DATA_BLOCK DB 10
VERSION : 0.1


  STRUCT
   Daten : ARRAY  [0 .. 255 ] OF BYTE ;
  END_STRUCT ;
BEGIN
   Daten[0] := B#16#0;
   Daten[1] := B#16#0;
   Daten[2] := B#16#0;
   Daten[3] := B#16#0;
   Daten[4] := B#16#0;
   Daten[5] := B#16#0;
   Daten[6] := B#16#0;
   Daten[7] := B#16#0;
   Daten[8] := B#16#0;
   Daten[9] := B#16#0;
   Daten[10] := B#16#0;
   Daten[11] := B#16#0;
   Daten[12] := B#16#0;
   Daten[13] := B#16#0;
   Daten[14] := B#16#0;
   Daten[15] := B#16#0;
   Daten[16] := B#16#0;
   Daten[17] := B#16#0;
   Daten[18] := B#16#0;
   Daten[19] := B#16#0;
   Daten[20] := B#16#0;
   Daten[21] := B#16#0;
   Daten[22] := B#16#0;
   Daten[23] := B#16#0;
   Daten[24] := B#16#0;
   Daten[25] := B#16#0;
   Daten[26] := B#16#0;
   Daten[27] := B#16#0;
   Daten[28] := B#16#0;
   Daten[29] := B#16#0;
   Daten[30] := B#16#0;
   Daten[31] := B#16#0;
   Daten[32] := B#16#0;
   Daten[33] := B#16#0;
   Daten[34] := B#16#0;
   Daten[35] := B#16#0;
   Daten[36] := B#16#0;
   Daten[37] := B#16#0;
   Daten[38] := B#16#0;
   Daten[39] := B#16#0;
   Daten[40] := B#16#0;
   Daten[41] := B#16#0;
   Daten[42] := B#16#0;
   Daten[43] := B#16#0;
   Daten[44] := B#16#0;
   Daten[45] := B#16#0;
   Daten[46] := B#16#0;
   Daten[47] := B#16#0;
   Daten[48] := B#16#0;
   Daten[49] := B#16#0;
   Daten[50] := B#16#0;
   Daten[51] := B#16#0;
   Daten[52] := B#16#0;
   Daten[53] := B#16#0;
   Daten[54] := B#16#0;
   Daten[55] := B#16#0;
   Daten[56] := B#16#0;
   Daten[57] := B#16#0;
   Daten[58] := B#16#0;
   Daten[59] := B#16#0;
   Daten[60] := B#16#0;
   Daten[61] := B#16#0;
   Daten[62] := B#16#0;
   Daten[63] := B#16#0;
   Daten[64] := B#16#0;
   Daten[65] := B#16#0;
   Daten[66] := B#16#0;
   Daten[67] := B#16#0;
   Daten[68] := B#16#0;
   Daten[69] := B#16#0;
   Daten[70] := B#16#0;
   Daten[71] := B#16#0;
   Daten[72] := B#16#0;
   Daten[73] := B#16#0;
   Daten[74] := B#16#0;
   Daten[75] := B#16#0;
   Daten[76] := B#16#0;
   Daten[77] := B#16#0;
   Daten[78] := B#16#0;
   Daten[79] := B#16#0;
   Daten[80] := B#16#0;
   Daten[81] := B#16#0;
   Daten[82] := B#16#0;
   Daten[83] := B#16#0;
   Daten[84] := B#16#0;
   Daten[85] := B#16#0;
   Daten[86] := B#16#0;
   Daten[87] := B#16#0;
   Daten[88] := B#16#0;
   Daten[89] := B#16#0;
   Daten[90] := B#16#0;
   Daten[91] := B#16#0;
   Daten[92] := B#16#0;
   Daten[93] := B#16#0;
   Daten[94] := B#16#0;
   Daten[95] := B#16#0;
   Daten[96] := B#16#0;
   Daten[97] := B#16#0;
   Daten[98] := B#16#0;
   Daten[99] := B#16#0;
   Daten[100] := B#16#0;
   Daten[101] := B#16#0;
   Daten[102] := B#16#0;
   Daten[103] := B#16#0;
   Daten[104] := B#16#0;
   Daten[105] := B#16#0;
   Daten[106] := B#16#0;
   Daten[107] := B#16#0;
   Daten[108] := B#16#0;
   Daten[109] := B#16#0;
   Daten[110] := B#16#0;
   Daten[111] := B#16#0;
   Daten[112] := B#16#0;
   Daten[113] := B#16#0;
   Daten[114] := B#16#0;
   Daten[115] := B#16#0;
   Daten[116] := B#16#0;
   Daten[117] := B#16#0;
   Daten[118] := B#16#0;
   Daten[119] := B#16#0;
   Daten[120] := B#16#0;
   Daten[121] := B#16#0;
   Daten[122] := B#16#0;
   Daten[123] := B#16#0;
   Daten[124] := B#16#0;
   Daten[125] := B#16#0;
   Daten[126] := B#16#0;
   Daten[127] := B#16#0;
   Daten[128] := B#16#0;
   Daten[129] := B#16#0;
   Daten[130] := B#16#0;
   Daten[131] := B#16#0;
   Daten[132] := B#16#0;
   Daten[133] := B#16#0;
   Daten[134] := B#16#0;
   Daten[135] := B#16#0;
   Daten[136] := B#16#0;
   Daten[137] := B#16#0;
   Daten[138] := B#16#0;
   Daten[139] := B#16#0;
   Daten[140] := B#16#0;
   Daten[141] := B#16#0;
   Daten[142] := B#16#0;
   Daten[143] := B#16#0;
   Daten[144] := B#16#0;
   Daten[145] := B#16#0;
   Daten[146] := B#16#0;
   Daten[147] := B#16#0;
   Daten[148] := B#16#0;
   Daten[149] := B#16#0;
   Daten[150] := B#16#0;
   Daten[151] := B#16#0;
   Daten[152] := B#16#0;
   Daten[153] := B#16#0;
   Daten[154] := B#16#0;
   Daten[155] := B#16#0;
   Daten[156] := B#16#0;
   Daten[157] := B#16#0;
   Daten[158] := B#16#0;
   Daten[159] := B#16#0;
   Daten[160] := B#16#0;
   Daten[161] := B#16#0;
   Daten[162] := B#16#0;
   Daten[163] := B#16#0;
   Daten[164] := B#16#0;
   Daten[165] := B#16#0;
   Daten[166] := B#16#0;
   Daten[167] := B#16#0;
   Daten[168] := B#16#0;
   Daten[169] := B#16#0;
   Daten[170] := B#16#0;
   Daten[171] := B#16#0;
   Daten[172] := B#16#0;
   Daten[173] := B#16#0;
   Daten[174] := B#16#0;
   Daten[175] := B#16#0;
   Daten[176] := B#16#0;
   Daten[177] := B#16#0;
   Daten[178] := B#16#0;
   Daten[179] := B#16#0;
   Daten[180] := B#16#0;
   Daten[181] := B#16#0;
   Daten[182] := B#16#0;
   Daten[183] := B#16#0;
   Daten[184] := B#16#0;
   Daten[185] := B#16#0;
   Daten[186] := B#16#0;
   Daten[187] := B#16#0;
   Daten[188] := B#16#0;
   Daten[189] := B#16#0;
   Daten[190] := B#16#0;
   Daten[191] := B#16#0;
   Daten[192] := B#16#0;
   Daten[193] := B#16#0;
   Daten[194] := B#16#0;
   Daten[195] := B#16#0;
   Daten[196] := B#16#0;
   Daten[197] := B#16#0;
   Daten[198] := B#16#0;
   Daten[199] := B#16#0;
   Daten[200] := B#16#0;
   Daten[201] := B#16#0;
   Daten[202] := B#16#0;
   Daten[203] := B#16#0;
   Daten[204] := B#16#0;
   Daten[205] := B#16#0;
   Daten[206] := B#16#0;
   Daten[207] := B#16#0;
   Daten[208] := B#16#0;
   Daten[209] := B#16#0;
   Daten[210] := B#16#0;
   Daten[211] := B#16#0;
   Daten[212] := B#16#0;
   Daten[213] := B#16#0;
   Daten[214] := B#16#0;
   Daten[215] := B#16#0;
   Daten[216] := B#16#0;
   Daten[217] := B#16#0;
   Daten[218] := B#16#0;
   Daten[219] := B#16#0;
   Daten[220] := B#16#0;
   Daten[221] := B#16#0;
   Daten[222] := B#16#0;
   Daten[223] := B#16#0;
   Daten[224] := B#16#0;
   Daten[225] := B#16#0;
   Daten[226] := B#16#0;
   Daten[227] := B#16#0;
   Daten[228] := B#16#0;
   Daten[229] := B#16#0;
   Daten[230] := B#16#0;
   Daten[231] := B#16#0;
   Daten[232] := B#16#0;
   Daten[233] := B#16#0;
   Daten[234] := B#16#0;
   Daten[235] := B#16#0;
   Daten[236] := B#16#0;
   Daten[237] := B#16#0;
   Daten[238] := B#16#0;
   Daten[239] := B#16#0;
   Daten[240] := B#16#0;
   Daten[241] := B#16#0;
   Daten[242] := B#16#0;
   Daten[243] := B#16#0;
   Daten[244] := B#16#0;
   Daten[245] := B#16#0;
   Daten[246] := B#16#0;
   Daten[247] := B#16#0;
   Daten[248] := B#16#0;
   Daten[249] := B#16#0;
   Daten[250] := B#16#0;
   Daten[251] := B#16#0;
   Daten[252] := B#16#0;
   Daten[253] := B#16#0;
   Daten[254] := B#16#0;
   Daten[255] := B#16#0;
END_DATA_BLOCK

DATA_BLOCK DB 11
VERSION : 0.1


  STRUCT
   Daten : ARRAY  [0 .. 255 ] OF BYTE ;
  END_STRUCT ;
BEGIN
   Daten[0] := B#16#0;
   Daten[1] := B#16#0;
   Daten[2] := B#16#0;
   Daten[3] := B#16#0;
   Daten[4] := B#16#0;
   Daten[5] := B#16#0;
   Daten[6] := B#16#0;
   Daten[7] := B#16#0;
   Daten[8] := B#16#0;
   Daten[9] := B#16#0;
   Daten[10] := B#16#0;
   Daten[11] := B#16#0;
   Daten[12] := B#16#0;
   Daten[13] := B#16#0;
   Daten[14] := B#16#0;
   Daten[15] := B#16#0;
   Daten[16] := B#16#0;
   Daten[17] := B#16#0;
   Daten[18] := B#16#0;
   Daten[19] := B#16#0;
   Daten[20] := B#16#0;
   Daten[21] := B#16#0;
   Daten[22] := B#16#0;
   Daten[23] := B#16#0;
   Daten[24] := B#16#0;
   Daten[25] := B#16#0;
   Daten[26] := B#16#0;
   Daten[27] := B#16#0;
   Daten[28] := B#16#0;
   Daten[29] := B#16#0;
   Daten[30] := B#16#0;
   Daten[31] := B#16#0;
   Daten[32] := B#16#0;
   Daten[33] := B#16#0;
   Daten[34] := B#16#0;
   Daten[35] := B#16#0;
   Daten[36] := B#16#0;
   Daten[37] := B#16#0;
   Daten[38] := B#16#0;
   Daten[39] := B#16#0;
   Daten[40] := B#16#0;
   Daten[41] := B#16#0;
   Daten[42] := B#16#0;
   Daten[43] := B#16#0;
   Daten[44] := B#16#0;
   Daten[45] := B#16#0;
   Daten[46] := B#16#0;
   Daten[47] := B#16#0;
   Daten[48] := B#16#0;
   Daten[49] := B#16#0;
   Daten[50] := B#16#0;
   Daten[51] := B#16#0;
   Daten[52] := B#16#0;
   Daten[53] := B#16#0;
   Daten[54] := B#16#0;
   Daten[55] := B#16#0;
   Daten[56] := B#16#0;
   Daten[57] := B#16#0;
   Daten[58] := B#16#0;
   Daten[59] := B#16#0;
   Daten[60] := B#16#0;
   Daten[61] := B#16#0;
   Daten[62] := B#16#0;
   Daten[63] := B#16#0;
   Daten[64] := B#16#0;
   Daten[65] := B#16#0;
   Daten[66] := B#16#0;
   Daten[67] := B#16#0;
   Daten[68] := B#16#0;
   Daten[69] := B#16#0;
   Daten[70] := B#16#0;
   Daten[71] := B#16#0;
   Daten[72] := B#16#0;
   Daten[73] := B#16#0;
   Daten[74] := B#16#0;
   Daten[75] := B#16#0;
   Daten[76] := B#16#0;
   Daten[77] := B#16#0;
   Daten[78] := B#16#0;
   Daten[79] := B#16#0;
   Daten[80] := B#16#0;
   Daten[81] := B#16#0;
   Daten[82] := B#16#0;
   Daten[83] := B#16#0;
   Daten[84] := B#16#0;
   Daten[85] := B#16#0;
   Daten[86] := B#16#0;
   Daten[87] := B#16#0;
   Daten[88] := B#16#0;
   Daten[89] := B#16#0;
   Daten[90] := B#16#0;
   Daten[91] := B#16#0;
   Daten[92] := B#16#0;
   Daten[93] := B#16#0;
   Daten[94] := B#16#0;
   Daten[95] := B#16#0;
   Daten[96] := B#16#0;
   Daten[97] := B#16#0;
   Daten[98] := B#16#0;
   Daten[99] := B#16#0;
   Daten[100] := B#16#0;
   Daten[101] := B#16#0;
   Daten[102] := B#16#0;
   Daten[103] := B#16#0;
   Daten[104] := B#16#0;
   Daten[105] := B#16#0;
   Daten[106] := B#16#0;
   Daten[107] := B#16#0;
   Daten[108] := B#16#0;
   Daten[109] := B#16#0;
   Daten[110] := B#16#0;
   Daten[111] := B#16#0;
   Daten[112] := B#16#0;
   Daten[113] := B#16#0;
   Daten[114] := B#16#0;
   Daten[115] := B#16#0;
   Daten[116] := B#16#0;
   Daten[117] := B#16#0;
   Daten[118] := B#16#0;
   Daten[119] := B#16#0;
   Daten[120] := B#16#0;
   Daten[121] := B#16#0;
   Daten[122] := B#16#0;
   Daten[123] := B#16#0;
   Daten[124] := B#16#0;
   Daten[125] := B#16#0;
   Daten[126] := B#16#0;
   Daten[127] := B#16#0;
   Daten[128] := B#16#0;
   Daten[129] := B#16#0;
   Daten[130] := B#16#0;
   Daten[131] := B#16#0;
   Daten[132] := B#16#0;
   Daten[133] := B#16#0;
   Daten[134] := B#16#0;
   Daten[135] := B#16#0;
   Daten[136] := B#16#0;
   Daten[137] := B#16#0;
   Daten[138] := B#16#0;
   Daten[139] := B#16#0;
   Daten[140] := B#16#0;
   Daten[141] := B#16#0;
   Daten[142] := B#16#0;
   Daten[143] := B#16#0;
   Daten[144] := B#16#0;
   Daten[145] := B#16#0;
   Daten[146] := B#16#0;
   Daten[147] := B#16#0;
   Daten[148] := B#16#0;
   Daten[149] := B#16#0;
   Daten[150] := B#16#0;
   Daten[151] := B#16#0;
   Daten[152] := B#16#0;
   Daten[153] := B#16#0;
   Daten[154] := B#16#0;
   Daten[155] := B#16#0;
   Daten[156] := B#16#0;
   Daten[157] := B#16#0;
   Daten[158] := B#16#0;
   Daten[159] := B#16#0;
   Daten[160] := B#16#0;
   Daten[161] := B#16#0;
   Daten[162] := B#16#0;
   Daten[163] := B#16#0;
   Daten[164] := B#16#0;
   Daten[165] := B#16#0;
   Daten[166] := B#16#0;
   Daten[167] := B#16#0;
   Daten[168] := B#16#0;
   Daten[169] := B#16#0;
   Daten[170] := B#16#0;
   Daten[171] := B#16#0;
   Daten[172] := B#16#0;
   Daten[173] := B#16#0;
   Daten[174] := B#16#0;
   Daten[175] := B#16#0;
   Daten[176] := B#16#0;
   Daten[177] := B#16#0;
   Daten[178] := B#16#0;
   Daten[179] := B#16#0;
   Daten[180] := B#16#0;
   Daten[181] := B#16#0;
   Daten[182] := B#16#0;
   Daten[183] := B#16#0;
   Daten[184] := B#16#0;
   Daten[185] := B#16#0;
   Daten[186] := B#16#0;
   Daten[187] := B#16#0;
   Daten[188] := B#16#0;
   Daten[189] := B#16#0;
   Daten[190] := B#16#0;
   Daten[191] := B#16#0;
   Daten[192] := B#16#0;
   Daten[193] := B#16#0;
   Daten[194] := B#16#0;
   Daten[195] := B#16#0;
   Daten[196] := B#16#0;
   Daten[197] := B#16#0;
   Daten[198] := B#16#0;
   Daten[199] := B#16#0;
   Daten[200] := B#16#0;
   Daten[201] := B#16#0;
   Daten[202] := B#16#0;
   Daten[203] := B#16#0;
   Daten[204] := B#16#0;
   Daten[205] := B#16#0;
   Daten[206] := B#16#0;
   Daten[207] := B#16#0;
   Daten[208] := B#16#0;
   Daten[209] := B#16#0;
   Daten[210] := B#16#0;
   Daten[211] := B#16#0;
   Daten[212] := B#16#0;
   Daten[213] := B#16#0;
   Daten[214] := B#16#0;
   Daten[215] := B#16#0;
   Daten[216] := B#16#0;
   Daten[217] := B#16#0;
   Daten[218] := B#16#0;
   Daten[219] := B#16#0;
   Daten[220] := B#16#0;
   Daten[221] := B#16#0;
   Daten[222] := B#16#0;
   Daten[223] := B#16#0;
   Daten[224] := B#16#0;
   Daten[225] := B#16#0;
   Daten[226] := B#16#0;
   Daten[227] := B#16#0;
   Daten[228] := B#16#0;
   Daten[229] := B#16#0;
   Daten[230] := B#16#0;
   Daten[231] := B#16#0;
   Daten[232] := B#16#0;
   Daten[233] := B#16#0;
   Daten[234] := B#16#0;
   Daten[235] := B#16#0;
   Daten[236] := B#16#0;
   Daten[237] := B#16#0;
   Daten[238] := B#16#0;
   Daten[239] := B#16#0;
   Daten[240] := B#16#0;
   Daten[241] := B#16#0;
   Daten[242] := B#16#0;
   Daten[243] := B#16#0;
   Daten[244] := B#16#0;
   Daten[245] := B#16#0;
   Daten[246] := B#16#0;
   Daten[247] := B#16#0;
   Daten[248] := B#16#0;
   Daten[249] := B#16#0;
   Daten[250] := B#16#0;
   Daten[251] := B#16#0;
   Daten[252] := B#16#0;
   Daten[253] := B#16#0;
   Daten[254] := B#16#0;
   Daten[255] := B#16#0;
END_DATA_BLOCK

DATA_BLOCK DB 99
VERSION : 0.1


  STRUCT
   Code1 : STRING  [30 ] := '123456789';
   Code2 : STRING  [30 ] := '1234567';
   Code3 : STRING  [30 ] := '09876542';
  END_STRUCT ;
BEGIN
   Code1 := '123456789';
   Code2 := '1234567';
   Code3 := '09876542';
END_DATA_BLOCK

FUNCTION_BLOCK FB 1
TITLE =
VERSION : 0.1


VAR_INPUT
  ScanCode : STRING  [50 ];
END_VAR
VAR
  Code1 : STRING  [50 ] := '4104450001085';
  Code2 : STRING  [50 ] := '4003240470004';
  Code3 : STRING  [50 ] := '4003240471001';
  Code4 : STRING  [50 ] := '4003240475009';
  Code5 : STRING  [50 ] := '4026843940262';
  Code6 : STRING  [50 ];
END_VAR
BEGIN
NETWORK
TITLE =

      CALL "EQ_STRNG" (
           S1                       := #ScanCode,
           S2                       := #Code1,
           RET_VAL                  := A      0.3);

      CALL "EQ_STRNG" (
           S1                       := #ScanCode,
           S2                       := #Code2,
           RET_VAL                  := A      0.4);



      CALL "EQ_STRNG" (
           S1                       := #ScanCode,
           S2                       := #Code3,
           RET_VAL                  := A      0.5);

      CALL "EQ_STRNG" (
           S1                       := #ScanCode,
           S2                       := #Code4,
           RET_VAL                  := A      0.6);


      CALL "EQ_STRNG" (
           S1                       := #ScanCode,
           S2                       := #Code5,
           RET_VAL                  := A      0.7);


      UN    A      0.3;
      UN    A      0.4;
      UN    A      0.5;
      UN    A      0.6;
      UN    A      0.7;
      =     A      0.1;


      L     #ScanCode[1];
      L     #ScanCode[2];
      L     #ScanCode[3];
      L     #ScanCode[4];
      L     #ScanCode[5];
      L     #ScanCode[6];
      L     #ScanCode[7];
      L     #ScanCode[8];
      L     #ScanCode[9];
      L     #ScanCode[10];
      L     #ScanCode[11];
      L     #ScanCode[12];
      L     #ScanCode[13];
      L     #ScanCode[14];
      L     #ScanCode[15];
      L     #ScanCode[16];


      L     #Code1[1];
      L     #Code1[2];
      L     #Code1[3];
      L     #Code1[4];
      L     #Code1[5];
      L     #Code1[6];
      L     #Code1[7];
      L     #Code1[8];
      L     #Code1[9];
      L     #Code1[10];
      L     #Code1[11];
      L     #Code1[12];










      BE    ;



END_FUNCTION_BLOCK

DATA_BLOCK DB 1
TITLE =
VERSION : 0.0

 FB 1
BEGIN
   ScanCode := '';
   Code1 := '4104450001085';
   Code2 := '4003240470004';
   Code3 := '4003240471001';
   Code4 := '4003240475009';
   Code5 := '4026843940262';
   Code6 := '';
END_DATA_BLOCK

FUNCTION_BLOCK FB 20
TITLE =RS 232 Schnittstelle
//S7-Baustein für die serielle Schnittstelle
//***************************************************************
VERSION : 0.1


VAR_INPUT
  Sende_DBNr : BLOCK_DB ;	//DB der die Sendedaten enthält
  Sende_ab_DWNr : INT ;	//Datenwortnummer ab dem die Sendedaten stehen
  Sende_Anzahl_Byte : INT ;	//Byteanzahl der Sendedaten
  Empfang_DBNr : BLOCK_DB ;	//DB der die Empfangsdaten enthält
  Empfang_ab_DWNr : INT ;	//Anfang Empfangsbuffer
  Empfang_Buf_Groesse : INT ;	//Groesse des Empfangsbuffers in BYTE (Umlaufbuffer)
  Eing_Doppelw : DWORD ;	//Eingangsdatendoppelwort der seriellen Klemme
END_VAR
VAR_OUTPUT
  Ausg_Doppelw : DWORD ;	//Ausgangsdatendoppelwort der seriellen Klemme
END_VAR
VAR_IN_OUT
  Empfang_naechstes_byte : INT ;	//Zeiger auf den naechsten Empfangsplatz im Umlaufbuffer
  RESET : BOOL ;	//Reset auf Schnittstelle
  SendeStart : BOOL ;	//Sendevorgang starten (wird nach vom Baustein geloescht)
END_VAR
VAR
  CONTROL : STRUCT 	//Controlbyte serial modul 750-65X
   TR : BOOL ;	//Sendeanforderung
   RA : BOOL ;	//Empfangsbestaetigung
   IR : BOOL ;	//Initialisierungsanforderung
   must_be_0 : BOOL ;	//always 0
   OL0 : BOOL ;	//Bytes available in input
   OL1 : BOOL ;	//Bytes available in input
   OL2 : BOOL ;	//Bytes available in input
   always_0 : BOOL ;	//always 0
  END_STRUCT ;
  Aus_Daten : DWORD ;
  Reset_aktiv : BOOL ;
  SendeNextByte : INT ;
  SendeAktiv : BOOL ;
  RestAnzahl : INT ;
END_VAR
VAR_TEMP
  E_Daten : ARRAY  [0 .. 2 ] OF BYTE ;
  STATUS : STRUCT 	//Statusbyte serial modul 750-65X
   TA : BOOL ;	//Uebertragungsbestaetigung
   RR : BOOL ;	//Empfangsanforderung
   IA : BOOL ;	//Initialisierungsbestaetigung
   BUF_F : BOOL ;	//Receiving buffer is full
   IL0 : BOOL ;	//Bytes available in input
   IL1 : BOOL ;	//Bytes available in input
   IL2 : BOOL ;	//Bytes available in input
   dummy : BOOL ;	//always 0
  END_STRUCT ;
  Index : BYTE ;
  Akt_Byte : BYTE ;
  AnzahlZeichen : BYTE ;
  Buffer_ende : INT ;
  SchiebeZahl : INT ;
END_VAR
BEGIN
NETWORK
TITLE =

//*******************************************************************************
//** STATUS-BYTE AUSFILTERN UND IN STRUKTUR SCHREIBEN ***************************
//*******************************************************************************
      L     #Eing_Doppelw; // Eingangswort einlesen
      SRD   16; // Statusbyte rechtsbuendig schieben
      LAR1  P##STATUS; // Anfangsadresse von der Variablen Status holen
      T     LB [AR1,P#0.0]; // Statusbyte in die Struktur schreiben
      SRW   4;
      L     B#16#7; // IL-Bit's einblenden
      UW    ;
      T     #AnzahlZeichen; // Anzahl verfügbarer Zeichen im Interface
//*******************************************************************************
//** EMPFANGSDATENBYTES IN ARRAY SCHREIBEN **************************************
//*******************************************************************************
      L     #Eing_Doppelw; // Eingangswort einlesen
      LAR1  P##E_Daten; // Anfangsadresse des E-Datenfeldes lesen
      T     LB [AR1,P#1.0]; // EB1 eintragen
      SRD   8;
      T     LB [AR1,P#2.0]; // EB2 eintragen
      SRD   16;
      T     LB [AR1,P#0.0]; // EB0 eintragen
//*******************************************************************************
//** ANFANGSWERTE SETZEN ********************************************************
//*******************************************************************************
      L     #Empfang_ab_DWNr;
      L     #Empfang_Buf_Groesse;
      +I    ;
      L     1;
      -I    ;
      T     #Buffer_ende;
      L     #Empfang_naechstes_byte;
      <I    ;
      SPB   SETZ;
      L     #Empfang_ab_DWNr;
      L     #Empfang_naechstes_byte;
      >I    ;
      SPB   SETZ;
      SPA   IO;
SETZ: L     #Empfang_ab_DWNr;
      T     #Empfang_naechstes_byte;
IO:   NOP   0;
//*******************************************************************************
NETWORK
TITLE =

//*******************************************************************************
//** INITIALISIEREN ???                              ****************************
//*******************************************************************************
      UN    #RESET;
      O     ;
      U     #Reset_aktiv;
      UN    #CONTROL.IR;
      UN    #STATUS.IA;
      SPB   NoRe; // No Reset
      U     #STATUS.IA;
      R     #CONTROL.IR;
      SPB   NoDa;
      U     #RESET;
      S     #Reset_aktiv;
      S     #CONTROL.IR;
      SPA   NoDa;
NoRe: U     #RESET;
      R     #RESET;
      R     #Reset_aktiv;
//*******************************************************************************
      U     #STATUS.RR; // Empfangsanforderung
      U     #CONTROL.RA; // Empfangsbestaetigung
      O     ;
      UN    #STATUS.RR; // Empfangsanforderung
      UN    #CONTROL.RA; // Empfangsbestaetigung
      SPB   NoDa; // Sprung 'KEINE DATEN DA'
//*******************************************************************************
//** DATEN DA UND ABHOLEN                            ****************************
//*******************************************************************************
      AUF   #Empfang_DBNr; // Empfangsdatenbaustein aufschlagen
      L     #E_Daten[0]; // 1.Datenbyte bearbeiten
      T     #Akt_Byte;
      L     0;
      T     #Index;
//*******************************************************************************
//** DATENBYTE UEBER POINTER IN DEN BUFFER SCHREIBEN ****************************
//** DO WHILE
//*******************************************************************************
NEXT: L     #Empfang_naechstes_byte; // Index naechster Bufferplatz
      SLD   3;
      L     DW#16#84000000; // Kennung DB einblenden
      OD    ; // in Pointerformat wandeln
      LAR1  ; // Adresse naechsten Bufferplatz laden
      L     #Akt_Byte; // Datenbyte
      T     B [AR1,P#0.0]; // in Buffer (Empfangs-DB) schreiben
//*******************************************************************************
//** INDEX AUF NAECHSTEN FREIEN SPEICHERPLATZ ERHOEHEN **************************
//*******************************************************************************
      L     #Empfang_naechstes_byte; // SPEICHER-INDEX erhoehen
      +     1;
      T     #Empfang_naechstes_byte;
      L     #Buffer_ende;
      <=I   ;
      SPB   OK;
      L     #Empfang_ab_DWNr;
      T     #Empfang_naechstes_byte;
OK:   NOP   0;
//*******************************************************************************
//** NAECHSTES VERFUEGBARES DATENBYTE HOLEN *************************************
//*******************************************************************************
      L     #E_Daten[1];
      T     #Akt_Byte;
      L     #Index;
      L     0;
      <=I   ;
      SPB   ZWEI;
      L     #E_Daten[2];
      T     #Akt_Byte;
ZWEI: NOP   0;
//*******************************************************************************
//** ALLE VERFUEGBAREN ZEICHEN ABGEARBEITET ? ***********************************
//*******************************************************************************
      L     #Index;
      L     1;
      +I    ;
      T     #Index;
      L     #AnzahlZeichen;
      <I    ;
      SPB   NEXT; // END DO WHILE
//*******************************************************************************
//** EMPFANG QUITTIEREN *********************************************************
//*******************************************************************************
      U     #STATUS.RR;
      =     #CONTROL.RA;
NoDa: NOP   1; //** EINSPRUNG WENN KEINE EMPFANGSDATEN DA
NETWORK
TITLE =

      U     #STATUS.TA; // Uebertragungsbestaetigung
      UN    #CONTROL.TR; // Sendeanforderung
      O     ;
      UN    #STATUS.TA; // Uebertragungsbestaetigung
      U     #CONTROL.TR; // Sendeanforderung
      O     ;
      UN    #SendeStart;
      SPB   NOTX; // Wenn keine Sendedaten dann Sprung
      U     #SendeAktiv;
      SPB   AKTV; // Wenn Senden aktiv Sprung
      L     #Sende_ab_DWNr; // sonst INITIALISIEREN
      T     #SendeNextByte;
      L     #Sende_Anzahl_Byte;
      T     #RestAnzahl;
AKTV: U     #SendeStart;
      S     #SendeAktiv;

      L     #RestAnzahl;
      L     0;
      <=I   ;
      R     #SendeStart;
      R     #SendeAktiv;
      SPB   NOTX; // SPRUNG WENN FERTIG MIT AUFTRAG

      AUF   #Sende_DBNr; // Sende-DB aufschlagen

      L     #Aus_Daten;
      L     DW#16#FF0000; // Alle Datenbytes auf Null setzen
      UD    ;
      T     #Aus_Daten;
      L     24;
      T     #SchiebeZahl;
      L     0;
      T     #AnzahlZeichen;
//*******************************************************************************
AGAN: L     #SendeNextByte; // Index naechstes Sendebyte
      SLD   3;
      L     DW#16#84000000; // Kennung DB einblenden
      OD    ;
      LAR1  ;

      L     #SchiebeZahl;
      L     B [AR1,P#0.0]; // Datenbyte aus DB holen
      SLD   ;
      L     #Aus_Daten;
      OD    ; // und in Ausgangsdaten blenden
      T     #Aus_Daten;
//*******************************************************************************
      L     #SendeNextByte; // Index naechstes Sendebyte
      L     1;
      +I    ;
      T     #SendeNextByte; // Index naechstes Sendebyte
      L     #AnzahlZeichen;
      L     1;
      +I    ;
      T     #AnzahlZeichen;
      L     #RestAnzahl;
      L     1;
      -I    ;
      T     #RestAnzahl;
      L     0;
      <=I   ;
      SPB   REDY;
      L     0;
      T     #SchiebeZahl;
      L     #AnzahlZeichen;
      L     2;
      <>I   ;
      SPB   EINS;
      L     8;
      T     #SchiebeZahl;

EINS: L     #AnzahlZeichen;
      L     3;
      <I    ;
      SPB   AGAN;
REDY: NOP   0;

      UN    #STATUS.TA; // Uebertragungsbestaetigung
      =     #CONTROL.TR; // Sendeanforderung

//*******************************************************************************
      U     #SendeAktiv;
      R     #CONTROL.OL0;
      R     #CONTROL.OL1;
      R     #CONTROL.OL2;
//*******************************************************************************
      L     #AnzahlZeichen;
      L     1;
      ==I   ;
      S     #CONTROL.OL0;
      R     #CONTROL.OL1;
      R     #CONTROL.OL2;
//*******************************************************************************
      L     #AnzahlZeichen;
      L     2;
      ==I   ;
      R     #CONTROL.OL0;
      S     #CONTROL.OL1;
      R     #CONTROL.OL2;
//*******************************************************************************
      L     #AnzahlZeichen;
      L     3;
      ==I   ;
      S     #CONTROL.OL0;
      S     #CONTROL.OL1;
      R     #CONTROL.OL2;
//*******************************************************************************




//*******************************************************************************





NOTX: NOP   0;
NETWORK
TITLE =


//*******************************************************************************
//** AUSGANGSDATEN ZUSAMMENSTELLEN UND AUSGEBEN *********************************
//*******************************************************************************
      LAR1  P##CONTROL;
      L     DIB [AR1,P#0.0];
      LAR1  P##Aus_Daten;
      T     DIB [AR1,P#1.0];
      L     #Aus_Daten;
      T     #Ausg_Doppelw;
//*******************************************************************************
      BE    ;
END_FUNCTION_BLOCK

DATA_BLOCK DB 20
TITLE =
VERSION : 0.0

 FB 20
BEGIN
   Sende_DBNr := DB 1;
   Sende_ab_DWNr := 0;
   Sende_Anzahl_Byte := 0;
   Empfang_DBNr := DB 1;
   Empfang_ab_DWNr := 0;
   Empfang_Buf_Groesse := 0;
   Eing_Doppelw := DW#16#0;
   Ausg_Doppelw := DW#16#0;
   Empfang_naechstes_byte := 0;
   RESET := FALSE;
   SendeStart := FALSE;
   CONTROL.TR := FALSE;
   CONTROL.RA := FALSE;
   CONTROL.IR := FALSE;
   CONTROL.must_be_0 := FALSE;
   CONTROL.OL0 := FALSE;
   CONTROL.OL1 := FALSE;
   CONTROL.OL2 := FALSE;
   CONTROL.always_0 := FALSE;
   Aus_Daten := DW#16#0;
   Reset_aktiv := FALSE;
   SendeNextByte := 0;
   SendeAktiv := FALSE;
   RestAnzahl := 0;
END_DATA_BLOCK

DATA_BLOCK DB 31
TITLE =
VERSION : 0.0

 FB 20
BEGIN
   Sende_DBNr := DB 1;
   Sende_ab_DWNr := 0;
   Sende_Anzahl_Byte := 0;
   Empfang_DBNr := DB 1;
   Empfang_ab_DWNr := 0;
   Empfang_Buf_Groesse := 0;
   Eing_Doppelw := DW#16#0;
   Ausg_Doppelw := DW#16#0;
   Empfang_naechstes_byte := 0;
   RESET := FALSE;
   SendeStart := FALSE;
   CONTROL.TR := FALSE;
   CONTROL.RA := FALSE;
   CONTROL.IR := FALSE;
   CONTROL.must_be_0 := FALSE;
   CONTROL.OL0 := FALSE;
   CONTROL.OL1 := FALSE;
   CONTROL.OL2 := FALSE;
   CONTROL.always_0 := FALSE;
   Aus_Daten := DW#16#0;
   Reset_aktiv := FALSE;
   SendeNextByte := 0;
   SendeAktiv := FALSE;
   RestAnzahl := 0;
END_DATA_BLOCK

FUNCTION_BLOCK FB 25
TITLE =
VERSION : 0.1


VAR_INPUT
  Startzeichen : BYTE ;
  Endezeichen : BYTE ;
  DB_Nr : BLOCK_DB ;
  Ab_Dw : INT ;
  Anzahl_Byte : INT ;
  Zeiger_Ende : INT ;
END_VAR
VAR_OUTPUT
  LetzterString : STRING  [50 ];
  Aenderung : BOOL ;
END_VAR
VAR
  alterAnfang : INT ;
END_VAR
VAR_TEMP
  Zeiger_akt_Byte : INT ;
  HilfsString : STRING  [50 ];
  Laenge : BYTE ;
  Ret_Value : INT ;
  Akt_Byte : BYTE ;
  Adresse : DWORD ;
END_VAR
BEGIN
NETWORK
TITLE =

//*******************************************************************************
//** SUCHZEIGER SETZEN                                ***************************
//*******************************************************************************
      L     #Zeiger_Ende;
      T     #Zeiger_akt_Byte;
      U     #Aenderung;
      R     #Aenderung;

      AUF   #DB_Nr;
//*******************************************************************************
//** ENDEZEICHEN SUCHEN                               ***************************
//*******************************************************************************
NEXT: NOP   1;

      L     #Zeiger_akt_Byte;
      L     1;
      -I    ;
      T     #Zeiger_akt_Byte;
      L     #Ab_Dw;
      >=I   ;
      SPB   OK;
      L     #Ab_Dw;
      L     #Anzahl_Byte;
      +I    ;
      L     1;
      -I    ;
      T     #Zeiger_akt_Byte;
OK:   NOP   1;
      L     #Zeiger_akt_Byte;
      L     #Zeiger_Ende;
      ==I   ;
      BEB   ;
      L     #Zeiger_akt_Byte;
      SLD   3;
      L     DW#16#84000000;
      OD    ;
      LAR1  ;
      L     B [AR1,P#0.0];
      L     #Endezeichen;
      <>I   ;
      SPB   NEXT;
//*******************************************************************************
//** STARTZEICHEN SUCHEN                              ***************************
//*******************************************************************************
NEX:  NOP   1;

      L     #Zeiger_akt_Byte;
      L     1;
      -I    ;
      T     #Zeiger_akt_Byte;
      L     #Ab_Dw;
      >=I   ;
      SPB   OK_2;
      L     #Ab_Dw;
      L     #Anzahl_Byte;
      +I    ;
      L     1;
      -I    ;
      T     #Zeiger_akt_Byte;
OK_2: NOP   1;
      L     #Zeiger_akt_Byte;
      L     #Zeiger_Ende;
      ==I   ;
      BEB   ;
      L     #Zeiger_akt_Byte;
      SLD   3;
      L     DW#16#84000000;
      OD    ;
      LAR1  ;
      L     B [AR1,P#0.0];
      L     #Startzeichen;
      <>I   ;
      SPB   NEX;
//*******************************************************************************
//** Zeichen umkopieren                               ***************************
//*******************************************************************************
      L     #Zeiger_akt_Byte;
      L     #alterAnfang;
      <>I   ;
      =     #Aenderung;
      L     #Zeiger_akt_Byte;
      T     #alterAnfang;
      L     0;
      T     #Laenge;

      LAR1  P##HilfsString;
      TAR1  #Adresse;
//*******************************************************************************
NEX1: L     #Zeiger_akt_Byte;
      L     1;
      +I    ;
      T     #Zeiger_akt_Byte;
      L     #Ab_Dw;
      L     #Anzahl_Byte;
      +I    ;
      L     #Zeiger_akt_Byte;
      >I    ;
      SPB   OK_1;
      L     #Ab_Dw;
      T     #Zeiger_akt_Byte;
OK_1: NOP   1;
//*******************************************************************************
      L     #Zeiger_akt_Byte;
      L     #Zeiger_Ende;
      ==I   ;
      BEB   ;
//*******************************************************************************
      L     #Zeiger_akt_Byte;
      SLD   3;
      L     DW#16#84000000;
      OD    ;
      LAR1  ;
      L     B [AR1,P#0.0];
      T     #Akt_Byte;
//*******************************************************************************
      L     #Akt_Byte;
      L     #Endezeichen;
      ==I   ;
      SPB   END;
//*******************************************************************************
      LAR1  #Adresse;
      L     #Akt_Byte;
      T     LB [AR1,P#2.0];
      +AR1  P#1.0;
      TAR1  #Adresse;
//*******************************************************************************
      L     #Laenge;
      L     1;
      +I    ;
      T     #Laenge;
      SPA   NEX1;
//*******************************************************************************
END:  NOP   1;

      LAR1  P##HilfsString;
      L     #Laenge;
      T     LB [AR1,P#1.0];
//*******************************************************************************
      CALL "BLKMOV" (
           SRCBLK                   := #HilfsString,
           RET_VAL                  := #Ret_Value,
           DSTBLK                   := #LetzterString);

      BE    ;

END_FUNCTION_BLOCK

DATA_BLOCK DB 25
TITLE =
VERSION : 0.0

 FB 25
BEGIN
   Startzeichen := B#16#0;
   Endezeichen := B#16#0;
   DB_Nr := DB 1;
   Ab_Dw := 0;
   Anzahl_Byte := 0;
   Zeiger_Ende := 0;
   LetzterString := '';
   Aenderung := FALSE;
   alterAnfang := 0;
END_DATA_BLOCK

FUNCTION_BLOCK FB 30
TITLE =
VERSION : 0.1


VAR_INPUT
  ScanCode : STRING  [50 ];
  SendeDB : BLOCK_DB ;
  Ab_DW : INT ;
END_VAR
VAR_OUTPUT
  StrLaenge : INT ;
END_VAR
VAR_TEMP
  Laenge : INT ;
  CopyByte : BYTE ;
END_VAR
BEGIN
NETWORK
TITLE =


      AUF   #SendeDB;

      CALL "LEN" (
           S                        := #ScanCode,
           RET_VAL                  := #Laenge);
      L     #Laenge;
      T     #StrLaenge;
      L     0;
      <=I   ;
      SPB   ENDE;

      L     #Laenge;
AGAN: T     #Laenge;

      L     P##ScanCode;
      LAR1  ;
      L     #Laenge;
      SLD   3;
      +AR1  ;
      L     DIB [AR1,P#1.0];
      T     #CopyByte;

      L     #Laenge;
      L     #Ab_DW;
      +I    ;
      L     1;
      -I    ;
      SLD   3;
      L     DW#16#84000000;
      OD    ;
      LAR1  ;
      L     #CopyByte;
      T     B [AR1,P#0.0];

      L     #Laenge;
      LOOP  AGAN;

ENDE: BE    ;



END_FUNCTION_BLOCK

DATA_BLOCK DB 30
TITLE =
VERSION : 0.0

 FB 30
BEGIN
   ScanCode := '';
   SendeDB := DB 1;
   Ab_DW := 0;
   StrLaenge := 0;
END_DATA_BLOCK

FUNCTION_BLOCK FB 100
TITLE =
VERSION : 0.1


VAR_INPUT
  Aenderung : BOOL ;
END_VAR
BEGIN
NETWORK
TITLE =
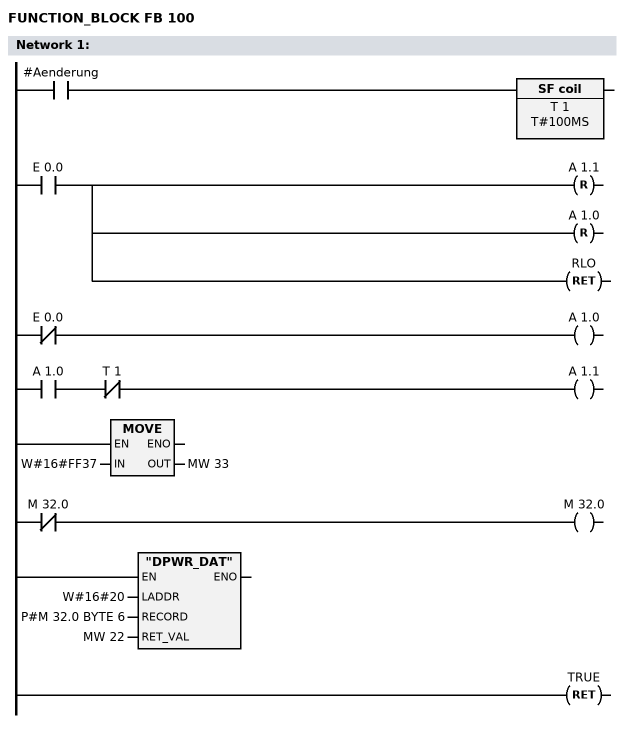
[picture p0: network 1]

      U     #Aenderung;
      L     T#100MS;
      SA    T      1;



      U     E      0.0;
      R     A      1.1;
      R     A      1.0;
      BEB   ;
      UN    E      0.0;
      =     A      1.0;
      U     A      1.0;
      UN    T      1;
      =     A      1.1;

      L     W#16#FF37;
      T     MW    33;
      UN    M     32.0;
      =     M     32.0;


      CALL "DPWR_DAT" (
           LADDR                    := W#16#20,
           RECORD                   := P#M 32.0 BYTE 6,
           RET_VAL                  := MW    22);





      BE    ;


END_FUNCTION_BLOCK

DATA_BLOCK DB 100
TITLE =
VERSION : 0.0

 FB 100
BEGIN
   Aenderung := FALSE;
END_DATA_BLOCK

ORGANIZATION_BLOCK OB 1
TITLE =
VERSION : 0.1


VAR_TEMP
  OB1_EV_CLASS : BYTE ;	//Bits 0-3 = 1 (Coming event), Bits 4-7 = 1 (Event class 1)
  OB1_SCAN_1 : BYTE ;	//1 (Cold restart scan 1 of OB 1), 3 (Scan 2-n of OB 1)
  OB1_PRIORITY : BYTE ;	//1 (Priority of 1 is lowest)
  OB1_OB_NUMBR : BYTE ;	//1 (Organization block 1, OB1)
  OB1_RESERVED_1 : BYTE ;	//Reserved for system
  OB1_RESERVED_2 : BYTE ;	//Reserved for system
  OB1_PREV_CYCLE : INT ;	//Cycle time of previous OB1 scan (milliseconds)
  OB1_MIN_CYCLE : INT ;	//Minimum cycle time of OB1 (milliseconds)
  OB1_MAX_CYCLE : INT ;	//Maximum cycle time of OB1 (milliseconds)
  OB1_DATE_TIME : DATE_AND_TIME ;	//Date and time OB1 started
  Empfangszeiger : INT ;
  Empfangszeiger02 : INT ;
  Start : BOOL ;
  DUMMY : DWORD ;
  Init : BOOL ;
  ScanCode : STRING  [50 ];
  Aenderung : BOOL ;
  Laenge : INT ;
END_VAR
BEGIN
NETWORK
TITLE =

// ********* RS232 IM SLAVE 3 BEDIENEN ********* //
// ** DATEN VON RS 232  IM SLAVE 3 ABHOLEN    ** //
// ** UND IM RINGBUFFER ABLEGEN               ** //
// ** AN DIESER SCHNITTSTELLE IST EIN SCANNER ** //
// ** ANGESCHLOSSEN.                          ** //
// ********************************************* //
      CALL FB    20 , DB    20 (
           Sende_DBNr               := DB    11,// SENDESPEICHER
           Sende_ab_DWNr            := 1,
           Sende_Anzahl_Byte        := #Laenge,
           Empfang_DBNr             := DB    10,// EMPFANGSBUFFER
           Empfang_ab_DWNr          := 1,
           Empfang_Buf_Groesse      := 30,
           Eing_Doppelw             := PED  256,
           Ausg_Doppelw             := PAD  256,
           Empfang_naechstes_byte   := #Empfangszeiger,// ZEIGT AUF NAECHSTEN FREIPLATZ IM RINGBUFFER
           RESET                    := M      0.0,// WIRD VOM TREIBER GELOESCHT
           SendeStart               := M      0.1);// WIRD VOM TREIBER GELOESCHT WENN ALLE ZEICHEN GESENDET


// ******************************************** //
// ** PROTOKOLLSTRING AUS RINGBUFFER SUCHEN  ** //
// ** DER SCANNER SENDET EIN ASCII-PROTOKOLL ** //
// **    STX   ASCII...  ETX                 ** //
// ******************************************** //
      CALL FB    25 , DB    25 (
           Startzeichen             := B#16#2,
           Endezeichen              := B#16#3,
           DB_Nr                    := DB    10,
           Ab_Dw                    := 1,
           Anzahl_Byte              := 30,
           Zeiger_Ende              := #Empfangszeiger,
           LetzterString            := #ScanCode,
           Aenderung                := #Aenderung);
// ******************************************** //

// ************************************************** //
// ** EINGESCANNTEN STRING IN SENDEBUFFER FUER DIE ** //
// ** RS 232 AM SLAVE 4 EINTRAGEN.                 ** //
// ************************************************** //
      CALL FB    30 , DB    30 (
           ScanCode                 := #ScanCode,
           SendeDB                  := DB    11,
           Ab_DW                    := 1,
           StrLaenge                := #Laenge);

// ************************************************** //
// ** EINGESCANNTEN STRING UEBER RS 232 AM SLAVE 4 ** //
// ** AUSGEBEN. AN DIESER SCHNITTSTELLE IST EIN PC ** //
// ** MIT EINEM TERMINALPROGRAMM ANGESCHLOSSEN     ** //
// ************************************************** //
      U     #Aenderung;
      S     #Start;

      CALL FB    20 , DB    31 (
           Sende_DBNr               := DB    11,
           Sende_ab_DWNr            := 1,
           Sende_Anzahl_Byte        := #Laenge,
           Empfang_DBNr             := DB    10,
           Empfang_ab_DWNr          := 100,
           Empfang_Buf_Groesse      := 10,
           Eing_Doppelw             := PED  260,
           Ausg_Doppelw             := PAD  260,
           Empfang_naechstes_byte   := #Empfangszeiger02,
           RESET                    := M      0.0,
           SendeStart               := #Start);




      CALL FB     1 , DB     1 (
           ScanCode                 := #ScanCode);

      CALL FB   100 , DB   100 (
           Aenderung                := #Aenderung);


      BE    ;
END_ORGANIZATION_BLOCK

